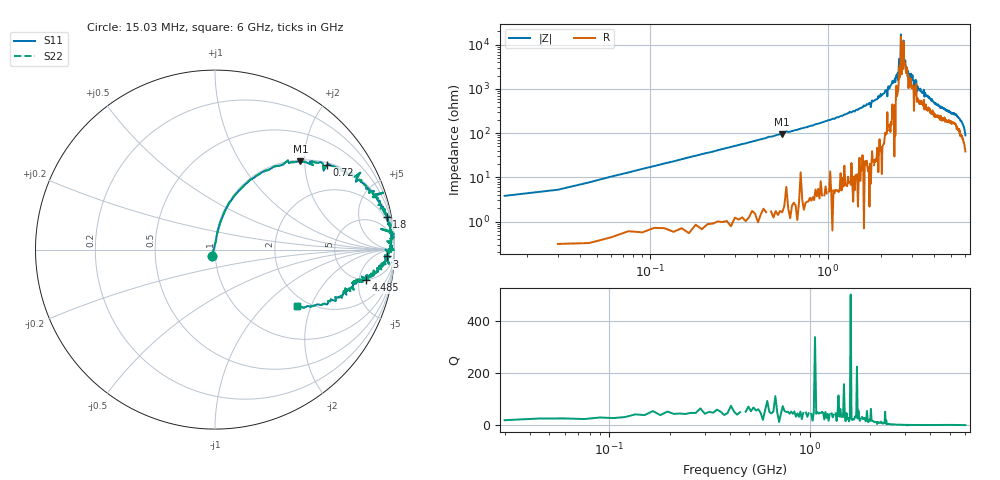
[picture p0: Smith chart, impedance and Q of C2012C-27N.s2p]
!	Network	Analyzer	HP8753E.07.74:	Oct	30	2002	Serial	No.	JP38451487
!	Hewlett-Packard
!	7	Sep	2009	10:49:08
!	Frequency	S11	S21	S12	S22
#	HZ	S	RI	R	50
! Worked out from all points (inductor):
!   400 points, 15.03 MHz to 6 GHz, reference 50 ohm
!   read as one part in series: L = 27.3 nH near 45.03 MHz
!   highest Q = 54.1 at 555 MHz (marker M1), where L = 27.3 nH
!   self-resonance near 2.58 GHz
!   S11 on the Smith chart (normalised r, x): 15.03 MHz: 0.97, -0.07; 720 MHz: 1.06, +2.59; 1.8 GHz: 1, +10; 3 GHz: 25, -24; 4.485 GHz: 4.87, -6.28; 6 GHz: 1.77, -1.60
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1.502992e7  -0.0163 -0.0344  1.02 0.0344  1.02 0.0344  -0.0163 -0.0344
1.650292e8  0.0787 0.26  0.921 -0.26  0.921 -0.26  0.0787 0.26
5.550272e8  0.476 0.491  0.524 -0.491  0.524 -0.491  0.476 0.491
7.200264e8  0.623 0.473  0.377 -0.473  0.377 -0.473  0.623 0.473
1.020025e9  0.789 0.396  0.211 -0.396  0.211 -0.396  0.789 0.396
1.800021e9  0.957 0.182  0.043 -0.182  0.043 -0.182  0.957 0.182
2.01002e9  0.971 0.137  0.0291 -0.137  0.0291 -0.137  0.971 0.137
2.505017e9  0.96 0.0464  0.0396 -0.0464  0.0396 -0.0464  0.96 0.0464
2.535017e9  0.987 0.0157  0.0133 -0.0157  0.0133 -0.0157  0.987 0.0157
2.580017e9  0.978 0.02  0.0224 -0.02  0.0224 -0.02  0.978 0.02
2.595017e9  0.995 -0.00256  0.00525 0.00256  0.00525 0.00256  0.995 -0.00256
2.625017e9  0.979 0.0223  0.021 -0.0223  0.021 -0.0223  0.979 0.0223
2.655017e9  0.966 -0.00162  0.0344 0.00162  0.0344 0.00162  0.966 -0.00162
2.685017e9  0.992 0.00232  0.00763 -0.00232  0.00763 -0.00232  0.992 0.00232
2.700016e9  0.976 0.00116  0.0243 -0.00116  0.0243 -0.00116  0.976 0.00116
2.775016e9  0.96 -0.00784  0.0403 0.00784  0.0403 0.00784  0.96 -0.00784
3.000015e9  0.959 -0.0384  0.0406 0.0384  0.0406 0.0384  0.959 -0.0384
3.015015e9  0.975 -0.0402  0.0252 0.0402  0.0252 0.0402  0.975 -0.0402
4.00501e9  0.884 -0.145  0.116 0.145  0.116 0.145  0.884 -0.145
4.485008e9  0.841 -0.17  0.159 0.17  0.159 0.17  0.841 -0.17
5.010005e9  0.782 -0.178  0.218 0.178  0.218 0.178  0.782 -0.178
6e9  0.458 -0.312  0.542 0.312  0.542 0.312  0.458 -0.312
